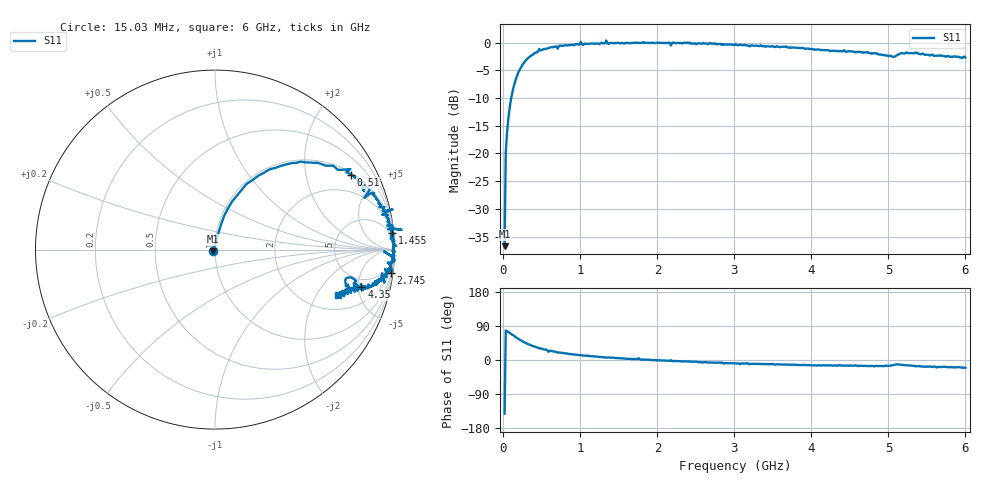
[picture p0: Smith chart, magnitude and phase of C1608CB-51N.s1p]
!	Network	Analyzer	HP8753E.07.74:	Oct	30	2002	Serial	No.	JP38451487
!	Hewlett-Packard
!	28	Aug	2009	8:16:16
!	Frequency	S11
#	HZ	S	RI	R	50
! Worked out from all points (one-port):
!   400 points, 15.03 MHz to 6 GHz, reference 50 ohm
!   lowest |S11| = -36.7 dB at 15.03 MHz (marker M1), VSWR 1.03, Z = 48.9 - j0.89 ohm
!   |S11| at or under -10 dB: start of sweep to 101.2 MHz
!   S11 on the Smith chart (normalised r, x): 15.03 MHz: 0.98, -0.02; 510 MHz: 1.10, +3.58; 1.455 GHz: 2, +21; 2.745 GHz: 1, -15; 4.35 GHz: 3.75, -5.39; 6 GHz: 2.84, -3.13
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1.502992e7  -0.0114 -0.0091
3.002985e7  0.0213 0.0993
6.00297e7  0.0517 0.189
1.050295e8  0.124 0.303
2.550287e8  0.429 0.482
4.650277e8  0.754 0.449
5.100274e8  0.756 0.416
5.850271e8  0.83 0.326
6.150269e8  0.828 0.375
7.650262e8  0.879 0.306
1.005025e9  0.99 0.224
1.035025e9  0.931 0.194
1.320023e9  0.979 0.121
1.335023e9  1.04 0.11
1.365023e9  0.964 0.115
1.455023e9  0.986 0.0909
1.515022e9  0.979 0.0781
2.145019e9  1 -0.0343
2.175019e9  0.942 -0.0104
2.265019e9  0.994 -0.05
2.745016e9  0.979 -0.128
3.015015e9  0.958 -0.152
3.765011e9  0.881 -0.19
4.350008e9  0.816 -0.209
4.515007e9  0.81 -0.21
5.040005e9  0.726 -0.186
5.265004e9  0.779 -0.202
6e9  0.687 -0.255
